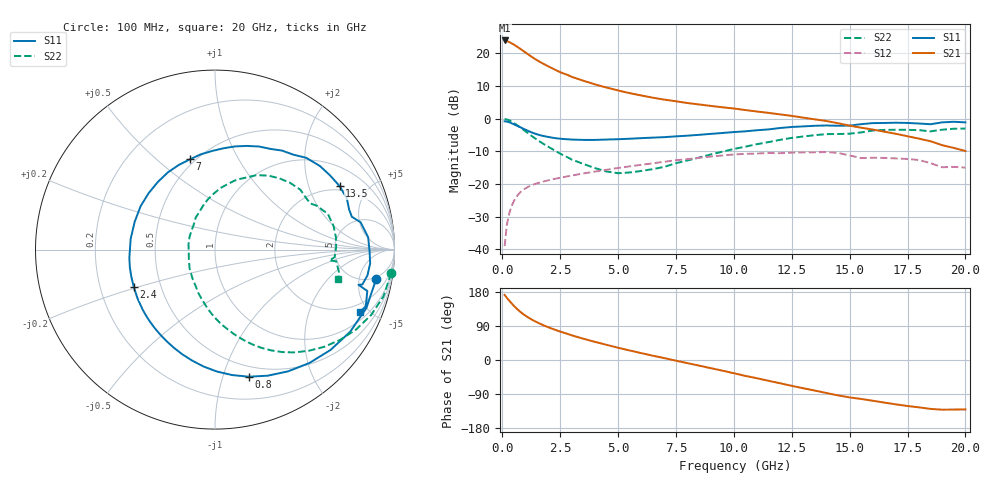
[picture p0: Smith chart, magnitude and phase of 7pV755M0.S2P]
! Infineon Technologies  Discrete & RF Semiconductors
! bfp620
! VCE = 0.75 V,  IC =  5.0 mA
! Common Emitter S-Parameters:  Sep 2002
# GHz  S  MA  R  50
!  f  S11  S21  S12  S22
! GHz  MAG  ANG  MAG  ANG  MAG  ANG  MAG  ANG
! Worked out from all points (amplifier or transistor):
!   59 points, 100 MHz to 20 GHz, reference 50 ohm
!   highest |S21| = 24.0 dB at 100 MHz (marker M1)
!   |S21| within 3 dB of that: start of sweep to 866.2 MHz
!   unconditionally stable (mu >= 1): 4.866 GHz to 11.46 GHz; 14.87 GHz to 15.27 GHz; 16.81 GHz to end of sweep
!   at 1 GHz: K = 0.32, MSG = 20.8 dB, |S12| = -21.3 dB
!   at 5.5 GHz: K = 1.04, MAG = 10.0 dB, |S12| = -14.6 dB
!   at 20 GHz: K = 1.58, MAG = -1.9 dB, |S12| = -15.0 dB
!   S11 on the Smith chart (normalised r, x): 100 MHz: 4.38, -8.70; 800 MHz: 0.40, -1.22; 2.4 GHz: 0.35, -0.19; 7 GHz: 0.47, +0.65; 13.5 GHz: 1.80, +3.24; 20 GHz: 1.43, -4.38
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0.1  0.9125 -10.5  15.76 171.7  0.0112 81.6  0.9902 -7.6
0.2  0.9039 -21.2  15.42 163.9  0.0241 78.6  0.9744 -15.5
0.3  0.8813 -31.3  14.89 156.5  0.0356 73.3  0.9433 -22.7
0.4  0.8525 -41.0  14.27 149.6  0.0458 68.2  0.9036 -29.5
0.5  0.8218 -50.3  13.6 143.0  0.0549 63.5  0.8597 -35.8
0.6  0.7912 -59.0  12.92 136.9  0.0629 59.3  0.8144 -41.7
0.8  0.7328 -75.1  11.58 126.1  0.0761 52.1  0.725 -52.2
0.9  0.7052 -82.3  10.94 121.3  0.0814 49.1  0.6823 -56.8
1.1  0.6543 -95.6  9.751 113.0  0.0901 44.0  0.6034 -64.9
1.3  0.611 -107.4  8.713 105.8  0.0969 40.0  0.5345 -71.8
1.5  0.577 -117.9  7.853 99.5  0.1026 36.9  0.4765 -78.0
1.9  0.5324 -136.0  6.564 88.6  0.1122 32.3  0.3881 -88.9
2.4  0.4984 -155.2  5.353 77.1  0.1227 28.1  0.3054 -101.2
2.8  0.485 -167.8  4.705 69.2  0.1308 25.4  0.2587 -111.1
3.5  0.4736 172.7  3.816 56.1  0.1452 20.8  0.2034 -128.2
5  0.4854 139.5  2.705 32.3  0.1761 11.2  0.1465 -174.9
7  0.5221 105.4  1.959 5.0  0.2192 -3.2  0.1834 130.0
8.5  0.5665 85.2  1.652 -14.8  0.2523 -16.1  0.2543 105.0
10.5  0.6411 61.0  1.357 -42.0  0.2897 -37.0  0.3733 78.8
13.5  0.7791 27.0  0.977 -80.7  0.3056 -67.9  0.5596 41.7
17  0.8679 -5.1  0.587 -117.1  0.2467 -98.2  0.6771 5.8
20  0.8785 -23.4  0.321 -130.3  0.1785 -112.6  0.7061 -13.4
